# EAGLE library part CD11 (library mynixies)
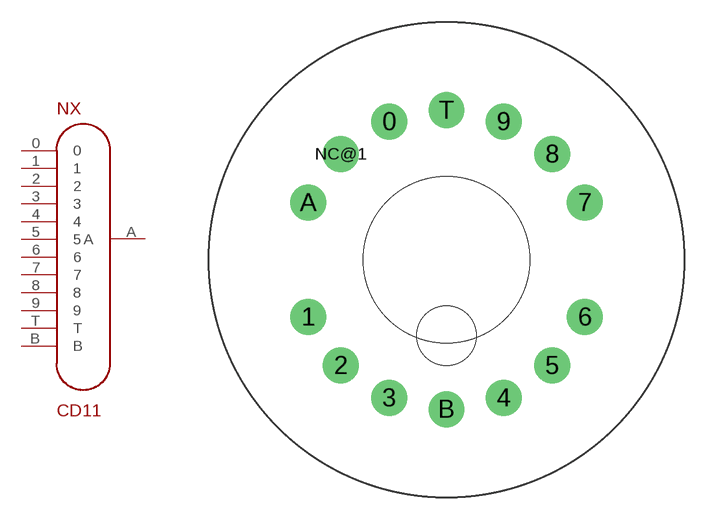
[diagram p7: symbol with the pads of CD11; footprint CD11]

Designator prefix NX

## CD11ALLPINS  [CD11]
0  0  pas
1  1  pas
2  2  pas
3  3  pas
4  4  pas
5  5  pas
6  6  pas
7  7  pas
8  8  pas
9  9  pas
A  A  pas
B  B  pas
T  T  pas

## Footprint CD11 (pad centres in mm)
drill 1.6: 0 -3.827,9.239; 1 -9.239,-3.827; 2 -7.071,-7.071; 3 -3.827,-9.239; 4 3.827,-9.239; 5 7.071,-7.071; 6 9.239,-3.827; 7 9.239,3.827; 8 7.071,7.071; 9 3.827,9.239; A -9.239,3.827; B 0,-10; NC@1 -7.071,7.071; T 0,10
hole 11.113 at 0,0
hole 3.969 at 0,-5.08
